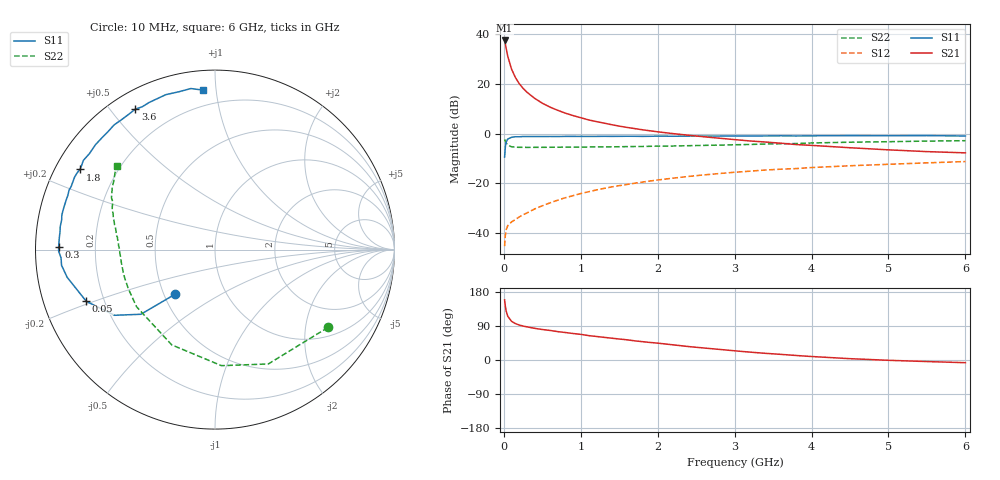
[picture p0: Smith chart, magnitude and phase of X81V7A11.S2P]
! SIEMENS Small Signal Semiconductors
! BFP136W
! Si NPN RF Bipolar Junction Transistor in SOT343
! VCE = 1.75 V  IC = 110 mA
! Common Emitter S-Parameters:  September  1994
# GHz  S  MA  R  50
!  f  S11  S21  S12  S22
! GHz  MAG  ANG  MAG  ANG  MAG  ANG  MAG  ANG
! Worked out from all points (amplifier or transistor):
!   40 points, 10 MHz to 6 GHz, reference 50 ohm
!   highest |S21| = 37.5 dB at 10 MHz (marker M1)
!   |S21| within 3 dB of that: start of sweep to 29.08 MHz
!   unconditionally stable (mu >= 1): 450.9 MHz to 2.955 GHz; 3.142 GHz to 3.234 GHz; 3.789 GHz to 3.813 GHz
!   at 200 MHz: K = 0.75, MSG = 26.8 dB, |S12| = -33.6 dB
!   at 1.5 GHz: K = 1.11, MAG = 10.0 dB, |S12| = -21.0 dB
!   at 6 GHz: K = 1.00, MSG = 1.7 dB, |S12| = -11.3 dB
!   S11 on the Smith chart (normalised r, x): 10 MHz: 0.57, -0.32; 50 MHz: 0.13, -0.19; 300 MHz: 0.07, +0.01; 1.8 GHz: 0.07, +0.27; 3.6 GHz: 0.07, +0.58; 6 GHz: 0.11, +0.92
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0.01  0.3352 -131.9  74.62 158.6  0.0054 66.3  0.7642 -34.6
0.02  0.5481 -138.9  62.86 141.3  0.009 56.2  0.703 -65.0
0.03  0.6683 -146.8  51.91 129.5  0.0115 46.5  0.6477 -86.8
0.05  0.7729 -158.1  36.31 115.8  0.0139 37.9  0.5831 -114.4
0.1  0.8382 -169.4  19.79 102.1  0.0166 36.8  0.5407 -143.9
0.15  0.8595 -174.2  13.42 96.1  0.0186 41.1  0.5299 -155.5
0.2  0.8589 -176.9  10.06 92.3  0.0209 43.9  0.5274 -161.8
0.25  0.8711 -179.4  8.121 89.5  0.0232 46.6  0.5272 -165.8
0.3  0.8713 179.1  6.784 87.5  0.0251 49.3  0.5259 -168.5
0.4  0.8699 175.6  5.108 83.6  0.0303 54.6  0.5268 -172.1
0.5  0.8692 173.4  4.073 80.5  0.0351 56.6  0.5275 -174.6
0.6  0.8718 171.5  3.398 78.0  0.0402 59.2  0.5285 -176.3
0.8  0.8748 167.3  2.568 72.5  0.051 61.3  0.531 -178.8
1.1  0.8739 161.3  1.881 64.4  0.0672 62.3  0.5353 178.4
1.4  0.875 156.3  1.505 57.6  0.084 61.5  0.5398 175.9
1.8  0.8749 149.3  1.19 48.4  0.1052 58.7  0.5482 172.7
2.2  0.8807 142.5  0.995 40.0  0.1263 55.5  0.5602 169.5
3.2  0.8916 125.7  0.708 20.8  0.1745 45.7  0.6021 160.6
3.6  0.8996 119.6  0.638 14.9  0.1911 41.7  0.6214 157.0
4.5  0.9057 107.6  0.517 3.5  0.2243 33.0  0.6681 149.0
5.5  0.9074 98.5  0.432 -4.1  0.2566 25.0  0.7037 142.3
6  0.8906 94.2  0.408 -7.1  0.2729 20.6  0.7171 139.3
